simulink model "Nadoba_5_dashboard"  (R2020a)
settings: Solver=VariableStepAuto  StartTime=0.0  StopTime=inf  RelTol=1e-3  EnableMultiTasking=on

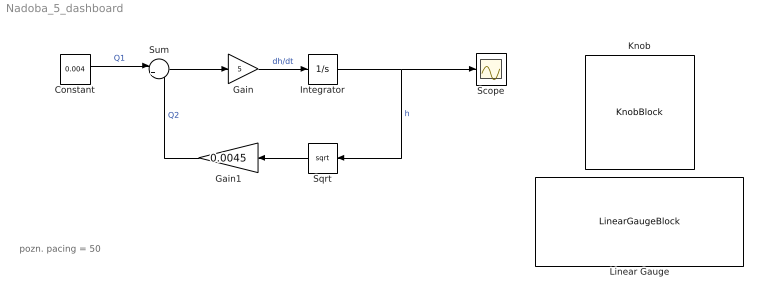
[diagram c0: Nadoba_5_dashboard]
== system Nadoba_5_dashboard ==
  note: pozn. pacing = 50
  Constant : Constant  Value=0.004
  Gain : Gain  Gain=5
  Gain1 : Gain  Gain=0.0045
  Integrator : Integrator  LimitOutput=on  UpperSaturationLimit=1
  Knob : KnobBlock  ScaleMax=0.005
  Linear Gauge : LinearGaugeBlock  ScaleMax=2
  Scope : Scope
  Sqrt : Sqrt
  Sum : Sum  Inputs=|+-
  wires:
  Gain/1 -> Integrator/1  "dh/dt"
  Constant/1 -> Sum/1  "Q1"
  Integrator/1 -> Scope/1, Sqrt/1  "h"
  Sqrt/1 -> Gain1/1
  Gain1/1 -> Sum/2  "Q2"
  Sum/1 -> Gain/1
